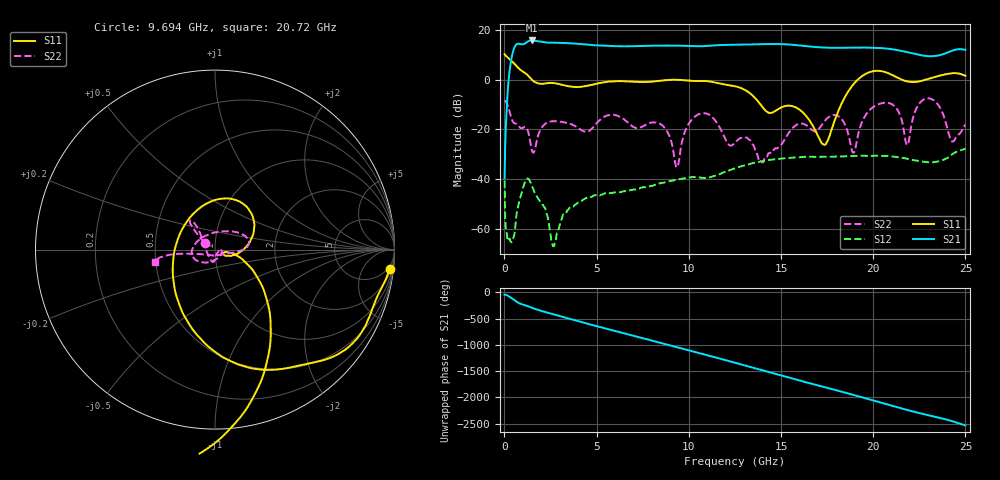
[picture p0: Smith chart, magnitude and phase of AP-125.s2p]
! MARKI MICROWAVE INC.
! Email:  info@markimicrowave.com  Phone:  408-778-4200
! Model Number:  AP-125  Date:  03/13
! Filename:		AP-125.S2P  Version: 1.0
! Description:  2-port S-parameter data for amplifier AP-125 measured at -20 dBm input power
! Frequency Measured: 	10 MHz to 25 GHz
! Measurements:		S11, S21, S12, S22
# Hz S  dB  R 50
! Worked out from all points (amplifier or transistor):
!   801 points, 10 MHz to 25 GHz, reference 50 ohm
!   highest |S21| = 15.7 dB at 1.478 GHz (marker M1)
!   |S21| within 3 dB of that: 530.9 MHz to 20.25 GHz (19.72 GHz wide, 190 % of centre)
!   unconditionally stable (mu >= 1): 1.535 GHz to 8.537 GHz; 10.03 GHz to 19 GHz; 21.89 GHz to 22.29 GHz
!   at 4.165 GHz: K = 12.68, MAG = 17.5 dB, |S12| = -48.7 dB
!   at 12.51 GHz: K = 2.77, MAG = 17.5 dB, |S12| = -35.6 dB
!   at 25 GHz: K = -1.09, MSG = 19.9 dB, |S12| = -27.8 dB
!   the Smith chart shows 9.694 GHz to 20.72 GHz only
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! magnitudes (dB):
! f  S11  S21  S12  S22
! 10 MHz  10.2  -39.6  -40.6  -8.3
! 228.7 MHz  8.6  0.0  -64.0  -11.5
! 447.3 MHz  7.1  10.8  -64.0  -16.8
! 1.072 GHz  2.9  14.3  -41.9  -19.0
! 1.478 GHz  0.0  15.7  -42.4  -28.0
! 2.665 GHz  -1.4  14.8  -66.9  -16.7
! 4.196 GHz  -2.8  14.3  -48.6  -20.3
! 8.35 GHz  -0.5  13.7  -41.7  -17.4
! 9.35 GHz  -0.1  13.6  -40.1  -35.2
! 10.6 GHz  -0.6  13.4  -39.2  -13.7
! 12.51 GHz  -2.7  14.0  -35.6  -25.3
! 13.94 GHz  -10.5  14.2  -32.8  -32.8
! 16.69 GHz  -18.1  13.2  -31.0  -20.3
! 17.44 GHz  -25.7  12.8  -31.0  -15.9
! 18.25 GHz  -10.1  12.8  -30.8  -15.6
! 18.94 GHz  -1.8  12.9  -30.7  -29.4
! 19.66 GHz  2.6  12.9  -30.6  -13.5
! 20.85 GHz  2.5  12.4  -30.7  -9.4
! 21.85 GHz  -0.7  11.0  -31.8  -26.3
! 22.84 GHz  0.0  9.5  -33.1  -7.6
! 24.28 GHz  2.6  11.6  -30.0  -24.8
! 25 GHz  1.5  12.0  -27.8  -18.0
